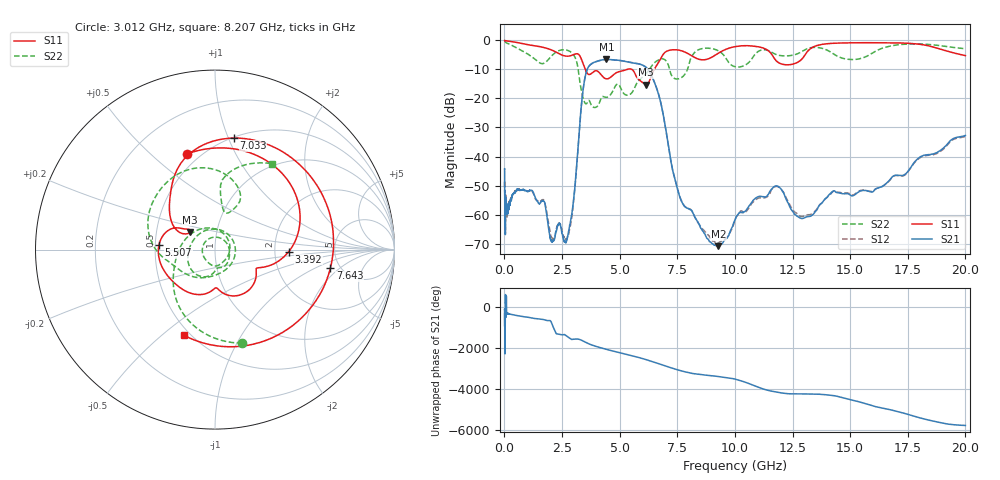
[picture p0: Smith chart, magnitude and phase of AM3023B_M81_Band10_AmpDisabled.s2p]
!Agilent Technologies,E8364B,MY43040894,A.07.50.67
!Agilent E8364B: A.07.50.67
!Date: Tuesday, October 27, 2020 10:41:15
!Correction: S11(Full 2 Port(1,2))
!S21(Full 2 Port(1,2))
!S12(Full 2 Port(1,2))
!S22(Full 2 Port(1,2))
!S2P File: Measurements: S11, S21, S12, S22:Log Frequency Sweep
# Hz S  dB  R 50
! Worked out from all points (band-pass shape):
!   3201 points, 10 MHz to 20 GHz, reference 50 ohm
!   highest |S21| = -6.79 dB at 4.426 GHz (marker M1); lowest = -70.7 dB at 9.286 GHz (marker M2)
!   |S21| within 3 dB of the highest: 3.615 GHz to 6.185 GHz (2.57 GHz wide, 52.4 % of centre)
!   lowest |S11| = -15.4 dB at 6.142 GHz (marker M3), VSWR 1.41, Z = 37.2 + j7.49 ohm
!   |S11| at or under -10 dB: 3.497 GHz to 5.44 GHz (1.943 GHz wide, 43.5 % of centre); 5.446 GHz to 6.516 GHz (1.07 GHz wide, 17.9 % of centre)
!   |S22| runs from -23.2 to -0.6 dB; largest |S21 - S12| = 0.0075
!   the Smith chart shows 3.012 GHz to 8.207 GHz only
!   S11 on the Smith chart (normalised r, x): 3.012 GHz: 0.43, +0.66; 3.392 GHz: 2.39, -0.06; 5.507 GHz: 0.52, +0.03; 7.033 GHz: 0.51, +1.05; 7.643 GHz: 4.17, -1.50; 8.207 GHz: 0.46, -0.59
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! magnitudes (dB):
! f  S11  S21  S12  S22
! 10 MHz  -0.3  -44.1  -50.5  -0.7
! 35.55 MHz  -0.4  -62.9  -63.8  -0.8
! 41.78 MHz  -0.4  -65.5  -64.6  -0.8
! 48.99 MHz  -0.4  -54.0  -53.9  -0.9
! 126.1 MHz  -0.5  -57.6  -58.5  -1.3
! 447.2 MHz  -0.8  -52.5  -52.0  -2.5
! 1.59 GHz  -2.5  -55.6  -55.2  -8.2
! 2.045 GHz  -3.5  -68.8  -67.6  -5.6
! 2.643 GHz  -5.6  -69.2  -68.4  -3.5
! 3.012 GHz  -5.1  -54.1  -54.9  -5.3
! 3.392 GHz  -7.7  -18.6  -18.6  -19.3
! 4.426 GHz  -13.4  -6.8  -6.8  -19.7
! 5.507 GHz  -10.1  -7.9  -7.9  -18.4
! 5.639 GHz  -11.2  -8.0  -8.0  -16.6
! 6.142 GHz  -15.4  -9.5  -9.4  -11.7
! 7.033 GHz  -4.0  -32.1  -32.2  -7.5
! 7.643 GHz  -3.7  -54.6  -54.3  -13.2
! 8.207 GHz  -5.9  -59.7  -59.7  -4.8
! 9.286 GHz  -4.6  -70.7  -69.6  -3.8
! 11.42 GHz  -3.6  -53.2  -53.7  -3.7
! 13.1 GHz  -4.5  -60.6  -60.0  -3.2
! 20 GHz  -5.5  -32.8  -33.1  -3.1
